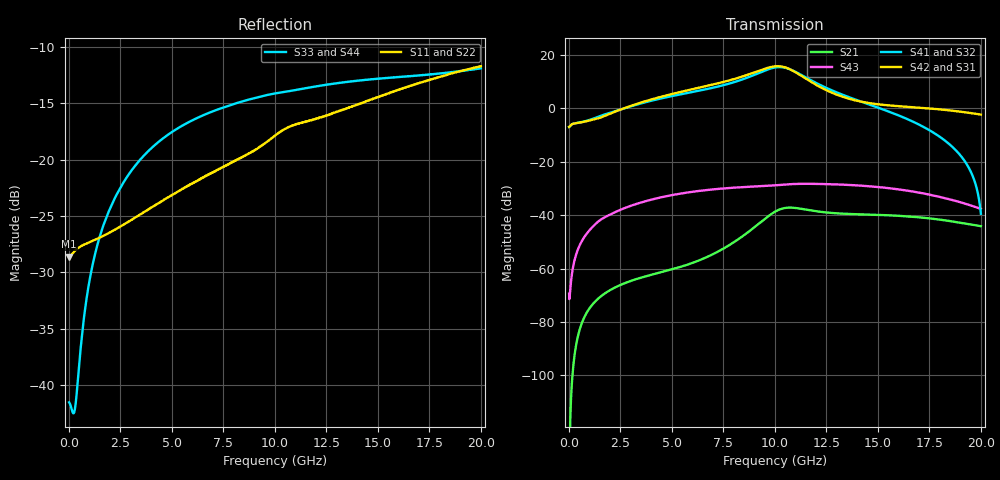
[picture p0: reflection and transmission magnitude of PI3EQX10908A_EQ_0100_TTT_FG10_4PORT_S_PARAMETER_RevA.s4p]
! NPort=4 DATA=2000 NOISE=0 GROUPDELAY=0 COMPLEX_DATAFORMAT=POLAR
! NumOfBlock=1 NumOfParam=0
! .MODEL Smodel S TSTONEFILE=PI3EQX10908A_EQ_0100_TTT_FG10_4PORT_S_PARAMETER_RevA.s4p TYPE=S
!  -- The above .MODEL line can be used for the S element in the netlist.
! The s parameter is extracted from the linear redriver, it is not bi-directional; only s(4,1)s(4,2) and s(3,1)s(3,2)
! should be the insertion loss
!Port definition:
!Port1 = input+
!Port2 = input-
!Port3 = output+
!Port4 = output-
# Hz S MA R  50
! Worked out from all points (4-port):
!   2000 points, 10 MHz to 20 GHz, reference 50 ohm
!   strongest paths, dB at 10 MHz, 5.01 GHz, 10.01 GHz, 15.01 GHz, 20 GHz:
!     S42: -6.9, 5.4, 15.8, 1.6, -2.3
!     S31: -6.9, 5.4, 15.8, 1.6, -2.3
!     S41: -6.9, 4.6, 15.4, 0.3, -39.4
!     S32: -6.9, 4.6, 15.4, 0.3, -39.4
!     S43: -69.4, -32.4, -28.8, -29.4, -37.6
!     S21: -127.2, -60.2, -38.7, -39.9, -44.1
!   lowest |S11| = -28.6 dB at 10 MHz (marker M1), VSWR 1.08, Z = 46.4 - j0.024 ohm
!   |S11| at or under -10 dB: start of sweep to end of sweep
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1e7  0.03701 -179.6  4.342e-07 14.4  0 0.0  0 0.0
     4.342e-07 14.4  0.03701 -179.6  0 0.0  0 0.0
     0.451 0.9  0.451 -179.1  0.008374 26.0  0.00034 -27.1
     0.451 -179.1  0.451 0.9  0.00034 -27.1  0.008374 26.0
7.78e9  0.0955 -117.2  0.002753 132.0  9.916e-07 51.6  4.176e-07 131.8
        0.002754 132.0  0.09554 -117.2  4.176e-07 131.8  9.916e-07 51.6
        3.345 -57.9  2.918 115.4  0.1737 3.4  0.03239 5.2
        2.918 115.4  3.345 -57.9  0.03239 5.2  0.1737 3.4
9.65e9  0.1205 -110.8  0.009407 115.1  4.025e-06 8.7  2.507e-06 119.7
        0.009408 115.1  0.1205 -110.8  2.507e-06 119.7  4.025e-06 8.7
        5.762 -111.8  5.367 62.7  0.1935 -10.4  0.03557 -13.0
        5.367 62.7  5.762 -111.8  0.03557 -13.0  0.1935 -10.4
1.056e10  0.1379 -111.5  0.01381 77.2  5.386e-06 -25.2  5.821e-06 82.8
          0.01381 77.2  0.138 -111.5  5.821e-06 82.8  5.386e-06 -25.2
          5.769 -160.8  5.702 12.1  0.2002 -16.4  0.03785 -22.4
          5.702 12.1  5.769 -160.9  0.03785 -22.4  0.2002 -16.4
1.153e10  0.1477 -112.9  0.01272 45.0  5.371e-06 -33.6  8.663e-06 45.1
          0.01272 45.0  0.1477 -112.9  8.663e-06 45.1  5.371e-06 -33.6
          3.548 160.7  3.751 -30.8  0.2074 -21.7  0.03881 -34.8
          3.751 -30.8  3.548 160.7  0.03881 -34.8  0.2074 -21.7
1.367e10  0.1708 -111.4  0.01055 15.4  1.397e-05 -38.6  1.725e-05 -4.4
          0.01055 15.4  0.1709 -111.4  1.725e-05 -4.4  1.397e-05 -38.6
          1.492 135.3  1.585 -77.2  0.2217 -32.6  0.03682 -60.8
          1.586 -77.2  1.492 135.3  0.03682 -60.8  0.2217 -32.6
2e10  0.2595 -114.2  0.006242 -43.8  9.112e-05 -147.7  7.23e-05 -137.3
      0.006242 -43.8  0.2596 -114.2  7.23e-05 -137.3  9.112e-05 -147.7
      0.7676 60.0  0.01067 -168.7  0.2539 -52.2  0.01317 -136.8
      0.01066 -168.7  0.7676 60.0  0.01317 -136.8  0.2539 -52.2
